//{{V2}}
FUNCTION_BLOCK FB98
TITLE=Set Enable State
//*****************************************************************************
//* maxon motor ag
//* R&D
//* all rights reserved
//*****************************************************************************
//* Summary:  Enable device
//*
//* Remarks:
//*
//* Created under: STEP7 REV5.2+SP1
//*****************************************************************************
//* History:
//* 18.05.2004 | INA   first release
//*
//*
//*****************************************************************************


AUTHOR:INA
FAMILY:StateMac
NAME:SetEnabl
VERSION:00.01


VAR_INPUT
       Write:BOOL //A rising edge start the command
       NodeID:BYTE //Adress of the maxon device
END_VAR

VAR_OUTPUT
       Done:BOOL //Data valid flag is TRUE if data were available
       Err:BOOL //Error flag is TRUE if an Error has occured, see ErrNo for more details
       ErrNo:DINT //Contains detailed error information
END_VAR

VAR_IN_OUT
END_VAR

VAR
       xEdgeMerker:BOOL //Edge Merker
       xEdgeFlag:BOOL //Edge Flag
       xStep:INT
       xShutdown:WORD:=W#16#0006
       xEnableOperation:WORD:=W#16#000F
END_VAR

VAR_TEMP
END_VAR
BEGIN

NETWORK
TITLE= Activate the service function
//{{a}}

// SDO Write "Set Enable State"

       U    #Write
       FP   #xEdgeFlag                   // recognize a positiv edge of the Read signal
       =    #xEdgeMerker                 // and set the xEdgeMerker for one cycle to true

       L    #xStep
       L    0
       ==I
       U    #xEdgeMerker
       SPB  nstp                         // iStep = 1 -> fnc1

       L    #xStep                       // jump list
       SPL  List
       SPA  rdef
       SPA  fnc1
       SPA  fnc2
       SPA  fncE
List  :SPA  rdef

rdef  :NOP  0
       R    #Done                        // reset Done
       R    #Err
       L    0
       T    #xStep                       // iStep = 0
       SPA  end

fnc1  :NOP  0
       CALL FC       15
         NodeID:=#NodeID
         Index:=DW#16#00006040
         SubIndex:=DW#16#00000000
         ValueIn:=#xShutdown
         RET_VAL:=#Done
         Err:=#Err
         ErrNo:=#ErrNo

       L    1
       U    #Err
       SPB  fncE

       SPA  nstp                         // iStep = 1 -> fnc2

fnc2  :NOP  0
       CALL FC       15
         NodeID:=#NodeID
         Index:=DW#16#00006040
         SubIndex:=DW#16#00000000
         ValueIn:=#xEnableOperation
         RET_VAL:=#Done
         Err:=#Err
         ErrNo:=#ErrNo

fncE  :NOP  0
       L    0
       T    #xStep
       SPA  end

nstp  :NOP  0
       L    #xStep
       INC            1
       T    #xStep

end   :NOP  0
END_FUNCTION_BLOCK
